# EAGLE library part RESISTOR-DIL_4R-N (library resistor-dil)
Array Chip Resistor Source: RS Component / Phycomp
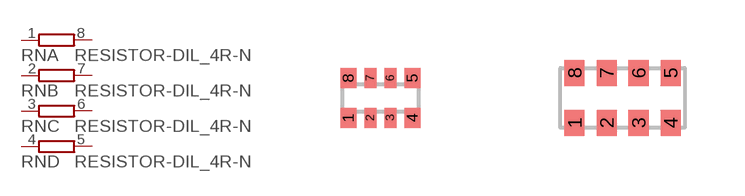
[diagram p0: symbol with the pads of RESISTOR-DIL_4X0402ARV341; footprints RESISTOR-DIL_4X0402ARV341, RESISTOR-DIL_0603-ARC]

Designator prefix RN; gates A=RESISTOR-DIL_R1NV B=RESISTOR-DIL_R1NV C=RESISTOR-DIL_R1NV D=RESISTOR-DIL_R1NV

## RESISTOR-DIL_4R-N0402ARV341  [RESISTOR-DIL_4X0402ARV341]
1  A:1  pas
2  B:1  pas
3  C:1  pas
4  D:1  pas
5  D:2  pas
6  C:2  pas
7  B:2  pas
8  A:2  pas

## RESISTOR-DIL_4R-N0603-ARC  [RESISTOR-DIL_0603-ARC]
Pads as for RESISTOR-DIL_4X0402ARV341

## RESISTOR-DIL_4R-N0603-ARV  [RESISTOR-DIL_0603-ARV]
Pads as for RESISTOR-DIL_4X0402ARV341

## RESISTOR-DIL_4R-NCAT16  [RESISTOR-DIL_CAT16]
Pads as for RESISTOR-DIL_4X0402ARV341

## RESISTOR-DIL_4R-NCAY16  [RESISTOR-DIL_CAY16]
Pads as for RESISTOR-DIL_4X0402ARV341

## RESISTOR-DIL_4R-NEXB18V  [RESISTOR-DIL_EXB18V]
Pads as for RESISTOR-DIL_4X0402ARV341

## RESISTOR-DIL_4R-NEXB28V  [RESISTOR-DIL_EXB28V]
Pads as for RESISTOR-DIL_4X0402ARV341

## RESISTOR-DIL_4R-NEXB38V  [RESISTOR-DIL_EXB38V]
Pads as for RESISTOR-DIL_4X0402ARV341

## RESISTOR-DIL_4R-NEXBN8V  [RESISTOR-DIL_EXBN8V]
Pads as for RESISTOR-DIL_4X0402ARV341

## RESISTOR-DIL_4R-NEXBS8V  [RESISTOR-DIL_EXBS8V]
Pads as for RESISTOR-DIL_4X0402ARV341

## RESISTOR-DIL_4R-NEXBV8V  [RESISTOR-DIL_EXBV8V]
Pads as for RESISTOR-DIL_4X0402ARV341

## RESISTOR-DIL_4R-NYC124  [RESISTOR-DIL_YC124]
Pads as for RESISTOR-DIL_4X0402ARV341

## Footprint RESISTOR-DIL_4X0402ARV341 (pad centres in mm)
Array chip resistor size 4 × 0402 Source: http://docs-europe.electrocomponents.com/webdocs/0114/0900766b80114d99.pdf
smd 0.4 x 0.5: 1 -0.8,-0.5; 4 0.8,-0.5; 5 0.8,0.5; 8 -0.8,0.5
smd 0.3 x 0.5: 2 -0.25,-0.5; 3 0.25,-0.5; 6 0.25,0.5; 7 -0.25,0.5

## Footprint RESISTOR-DIL_0603-ARC (pad centres in mm)
Chip Resistor Array size 4 × 0603 concave termination - Phycomp Components Source: RS Components
smd 0.5 x 0.65: 1 -1.2,-0.625; 2 -0.4,-0.625; 3 0.4,-0.625; 4 1.2,-0.625; 5 1.2,0.625; 6 0.4,0.625; 7 -0.4,0.625; 8 -1.2,0.625

## Footprint RESISTOR-DIL_0603-ARV (pad centres in mm)
Chip Resistor Array size 4 × 0603 convex termination - Phycomp Components Source: RS Components
smd 0.5 x 0.65: 1 -1.2,-0.625; 2 -0.4,-0.625; 3 0.4,-0.625; 4 1.2,-0.625; 5 1.2,0.625; 6 0.4,0.625; 7 -0.4,0.625; 8 -1.2,0.625

## Footprint RESISTOR-DIL_CAT16 (pad centres in mm)
BOURNS Chip Resistor Array Source: RS Component / BUORNS
smd 0.5 x 0.65: 1 -1.2,-0.675; 2 -0.4,-0.675; 3 0.4,-0.675; 4 1.2,-0.675; 5 1.2,0.675; 6 0.4,0.675; 7 -0.4,0.675; 8 -1.2,0.675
